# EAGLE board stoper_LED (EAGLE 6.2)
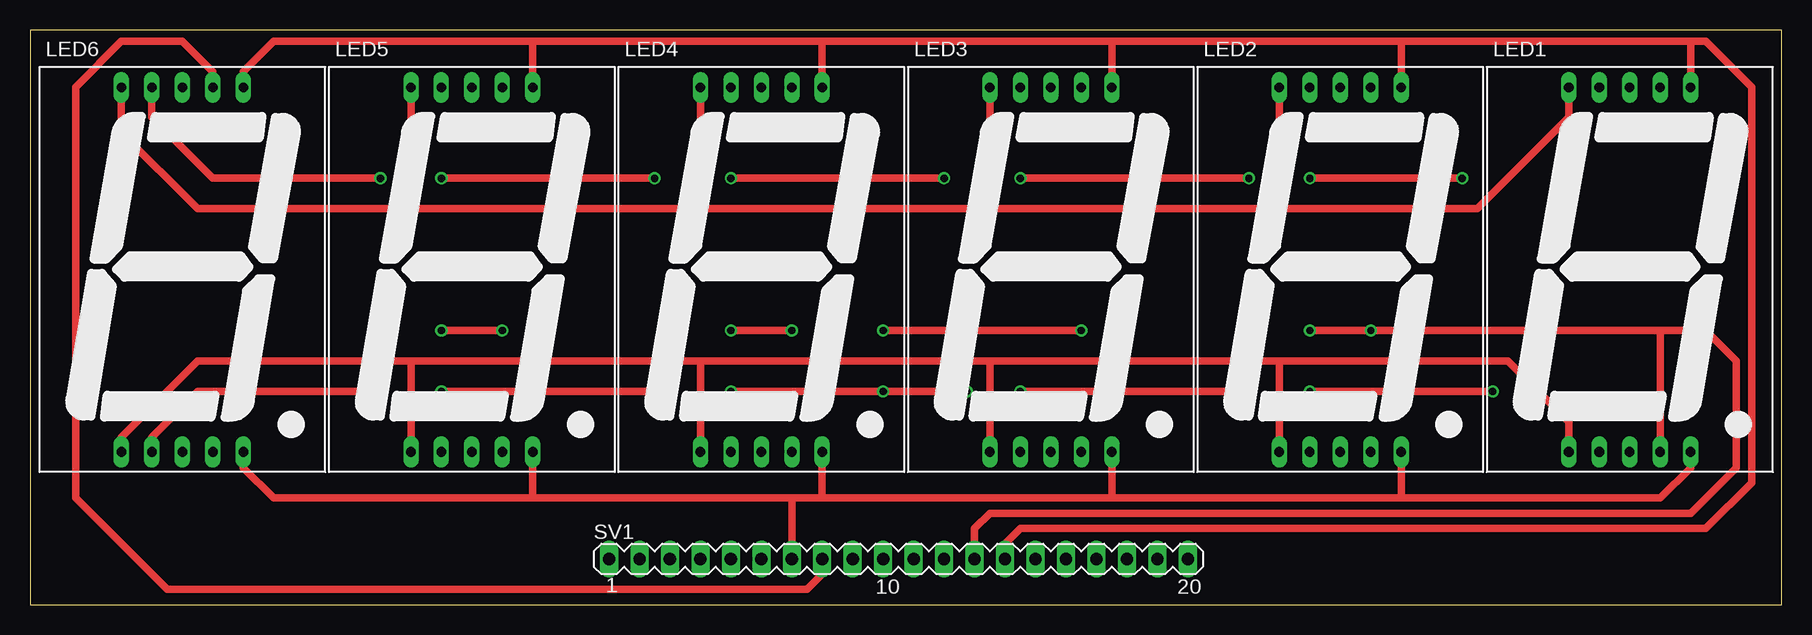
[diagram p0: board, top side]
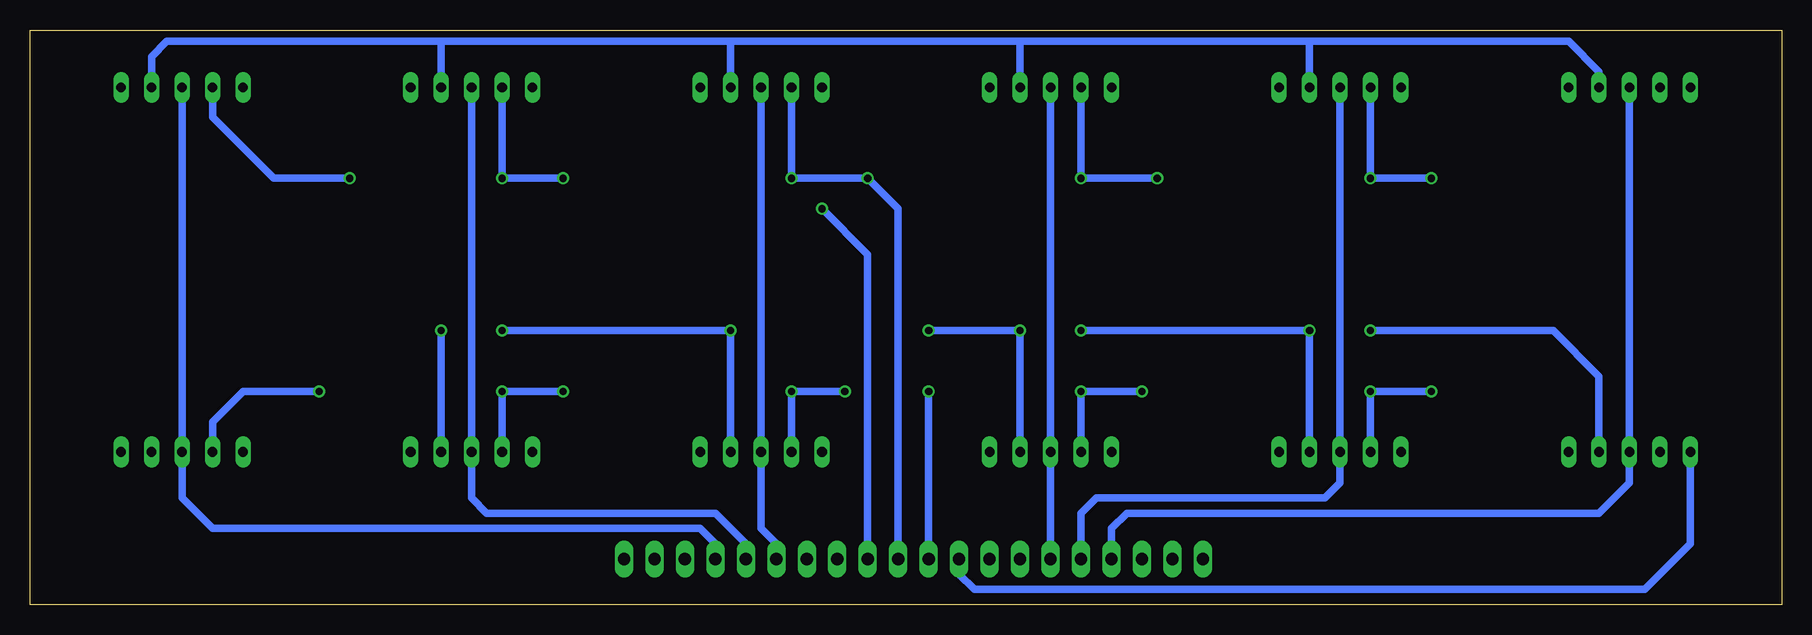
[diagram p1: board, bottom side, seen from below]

Size 146.03 x 47.93 mm. Coordinates in mm from the lower left corner, seen from the top.
Outline: 0,0 146.03,0 146.03,47.93 0,47.93 0,0
Copper layers (1*16): Top 0.035mm / dielectric 1.5mm / Bottom 0.035mm
Design rules: minimum track width 10mil, minimum drill 24mil, track to track 8mil, track to pad 8mil, pad to pad 8mil, via to via 8mil, smd to smd 8mil, copper to edge 40mil, drill to drill 8mil, minimum pad ring 10mil, minimum via ring 8mil, stop-mask expansion 4mil, vias tented up to drill 0mil, thermal gap 10mil

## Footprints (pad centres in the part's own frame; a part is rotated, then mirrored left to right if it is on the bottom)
SA10-21 = drill 0.8 long: 1 -5.08,-15.2; 2 -2.54,-15.2; 3 0,-15.2; 4 2.54,-15.2; 5 5.08,-15.2; 6 -5.08,15.2; 7 -2.54,15.2; 8 0,15.2; 9 2.54,15.2; 10 5.08,15.2
MA20-1 = drill 1.016 long: 1 -24.13,0; 2 -21.59,0; 3 -19.05,0; 4 -16.51,0; 5 -13.97,0; 6 -11.43,0; 7 -8.89,0; 8 -6.35,0; 9 -3.81,0; 10 -1.27,0; 11 1.27,0; 12 3.81,0; 13 6.35,0; 14 8.89,0; 15 11.43,0; 16 13.97,0; 17 16.51,0; 18 19.05,0; 19 21.59,0; 20 24.13,0

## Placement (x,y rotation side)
LED1  7-SEG_SA10-21  [SA10-21]  133.35,27.94 0 top
LED2  7-SEG_SA10-21  [SA10-21]  109.22,27.94 0 top
LED3  7-SEG_SA10-21  [SA10-21]  85.09,27.94 0 top
LED4  7-SEG_SA10-21  [SA10-21]  60.96,27.94 0 top
LED5  7-SEG_SA10-21  [SA10-21]  36.83,27.94 0 top
LED6  7-SEG_SA10-21  [SA10-21]  12.7,27.94 0 top
SV1  [MA20-1]  72.39,3.81 0 top

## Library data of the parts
LED1-LED6 = display-kingbright; OC_FARNELL: unknown; OC_NEWARK: unknown
SV1 = con-lstb; OC_FARNELL: unknown; OC_NEWARK: unknown

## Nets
A: LED1.7 LED2.7 LED3.7 LED4.7 LED5.7 LED6.7 SV1.11
B: LED1.6 LED2.6 LED3.6 LED4.6 LED5.6 LED6.6 SV1.12
C: LED1.4 LED2.4 LED3.4 LED4.4 LED5.4 LED6.4 SV1.13
D: LED1.2 LED2.2 LED3.2 LED4.2 LED5.2 LED6.2 SV1.10
DP: LED1.5 LED2.5 LED3.5 LED4.5 LED5.5 LED6.5 SV1.7
E: LED1.1 LED2.1 LED3.1 LED4.1 LED5.1 LED6.1 SV1.9
F: LED1.9 LED2.9 LED3.9 LED4.9 LED5.9 LED6.9 SV1.8
G: LED1.10 LED2.10 LED3.10 LED4.10 LED5.10 LED6.10 SV1.14
W1: LED1.3 LED1.8 SV1.17
W2: LED2.3 LED2.8 SV1.16
W3: LED3.3 LED3.8 SV1.15
W4: LED4.3 LED4.8 SV1.6
W5: LED5.3 LED5.8 SV1.5
W6: LED6.3 LED6.8 SV1.4

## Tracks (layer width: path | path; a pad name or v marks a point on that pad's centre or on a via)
A  (via drill 0.6)
  Top 0.61: LED6.7 10.16,40.64 15.24,35.56 v29.21,35.56 | v34.29,35.56 v52.07,35.56 | v58.42,35.56 v76.2,35.56 | v82.55,35.56 v101.6,35.56 | v106.68,35.56 v119.38,35.56
  Bottom 0.61: v29.21,35.56 v34.29,35.56 LED5.7 | v52.07,35.56 v58.42,35.56 LED4.7 | v101.6,35.56 v106.68,35.56 LED2.7 | v119.38,35.56 125.73,35.56 130.81,40.64 LED1.7 | LED3.7 v82.55,35.56 v76.2,35.56 73.66,33.02 SV1.11
B  (via drill 0.6)
  Top 0.61: LED6.6 7.62,39.37 13.97,33.02 31.75,33.02 | 31.75,33.02 55.88,33.02 | 55.88,33.02 v80.01,33.02 | v80.01,33.02 104.14,33.02 | 104.14,33.02 120.65,33.02 128.27,40.64 LED1.6 | LED2.6 104.14,33.02 | LED3.6 80.01,34.29 v80.01,33.02 | LED5.6 31.75,33.02 | LED4.6 55.88,33.02
  Bottom 0.61: SV1.12 76.2,29.21 v80.01,33.02
C  (via drill 0.6)
  Top 0.61: v34.29,22.86 v39.37,22.86 | v58.42,22.86 v63.5,22.86 | v71.12,22.86 v87.63,22.86 | v106.68,22.86 v111.76,22.86 135.89,22.86 | 135.89,22.86 LED1.4 | SV1.13 78.74,6.35 80.01,7.62 138.43,7.62 142.24,11.43 142.24,20.32 139.7,22.86 135.89,22.86
  Bottom 0.61: LED6.4 15.24,19.05 19.05,22.86 v34.29,22.86 | v58.42,22.86 v39.37,22.86 LED5.4 | v71.12,22.86 v63.5,22.86 LED4.4 | v106.68,22.86 v87.63,22.86 LED3.4 | LED2.4 v111.76,22.86
D  (via drill 0.6)
  Top 0.61: LED6.2 10.16,13.97 13.97,17.78 v29.21,17.78 | v34.29,17.78 v53.34,17.78 | v58.42,17.78 v71.12,17.78 v78.11,17.78 | v82.55,17.78 v101.6,17.78 | v106.68,17.78 v121.92,17.78
  Bottom 0.61: v29.21,17.78 v34.29,17.78 LED5.2 | v53.34,17.78 v58.42,17.78 LED4.2 | v78.11,17.78 v82.55,17.78 LED3.2 | v101.6,17.78 v106.68,17.78 LED2.2 | v121.92,17.78 128.27,17.78 130.81,15.24 LED1.2 | SV1.10 v71.12,17.78
DP
  Top 0.61: LED6.5 17.78,11.43 20.32,8.89 41.91,8.89 | 41.91,8.89 63.5,8.89 | 63.5,8.89 66.04,8.89 | 66.04,8.89 90.17,8.89 | 90.17,8.89 114.3,8.89 | 114.3,8.89 135.89,8.89 138.43,11.43 LED1.5 | LED2.5 114.3,8.89 | LED3.5 90.17,8.89 | LED4.5 66.04,8.89 | SV1.7 63.5,8.89 | LED5.5 41.91,8.89
E
  Top 0.61: LED6.1 7.62,13.97 13.97,20.32 31.75,20.32 | 31.75,20.32 55.88,20.32 | 55.88,20.32 80.01,20.32 | 80.01,20.32 104.14,20.32 | 104.14,20.32 123.19,20.32 128.27,15.24 LED1.1 | LED2.1 104.14,20.32 | LED3.1 80.01,20.32 | LED4.1 55.88,20.32 | LED5.1 31.75,20.32
  Bottom 0.61: LED6.1 7.62,5.08 11.43,1.27 67.31,1.27 68.58,2.54 SV1.9
F
  Top 0.61: SV1.8 66.04,2.54 64.77,1.27 11.43,1.27 3.81,8.89 3.81,43.18 7.62,46.99 12.7,46.99 15.24,44.45 LED6.9
  Bottom 0.61: LED1.9 135.89,45.72 134.62,46.99 111.76,46.99 | 111.76,46.99 87.63,46.99 | 87.63,46.99 63.5,46.99 | 63.5,46.99 39.37,46.99 | 39.37,46.99 17.78,46.99 15.24,44.45 LED6.9 | LED5.9 39.37,46.99 | LED4.9 63.5,46.99 | LED3.9 87.63,46.99 | LED2.9 111.76,46.99
G
  Top 0.61: LED4.10 66.04,46.99 | 66.04,46.99 90.17,46.99 | 90.17,46.99 114.3,46.99 | 114.3,46.99 138.43,46.99 | 138.43,46.99 LED1.10 | LED2.10 114.3,46.99 | LED3.10 90.17,46.99 | LED6.10 17.78,44.45 20.32,46.99 41.91,46.99 | 41.91,46.99 66.04,46.99 | LED5.10 41.91,46.99 | SV1.14 81.28,5.08 82.55,6.35 139.7,6.35 143.51,10.16 143.51,43.18 139.7,46.99 138.43,46.99
W1
  Bottom 0.61: SV1.17 88.9,5.08 90.17,6.35 130.81,6.35 133.35,8.89 LED1.3 LED1.8
W2
  Bottom 0.61: SV1.16 86.36,5.08 88.9,7.62 107.95,7.62 109.22,8.89 LED2.3 LED2.8
W3
  Bottom 0.61: SV1.15 83.82,5.08 85.09,6.35 LED3.3 LED3.8
W4
  Bottom 0.61: SV1.6 LED4.3 LED4.8
W5
  Bottom 0.61: LED5.8 LED5.3 36.83,10.16 38.1,8.89 57.15,8.89 58.42,7.62 SV1.5
W6
  Bottom 0.61: SV1.4 55.88,6.35 54.61,7.62 15.28,7.62 12.7,10.16 LED6.3 LED6.8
